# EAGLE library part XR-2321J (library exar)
V.23/V.21 MODEM
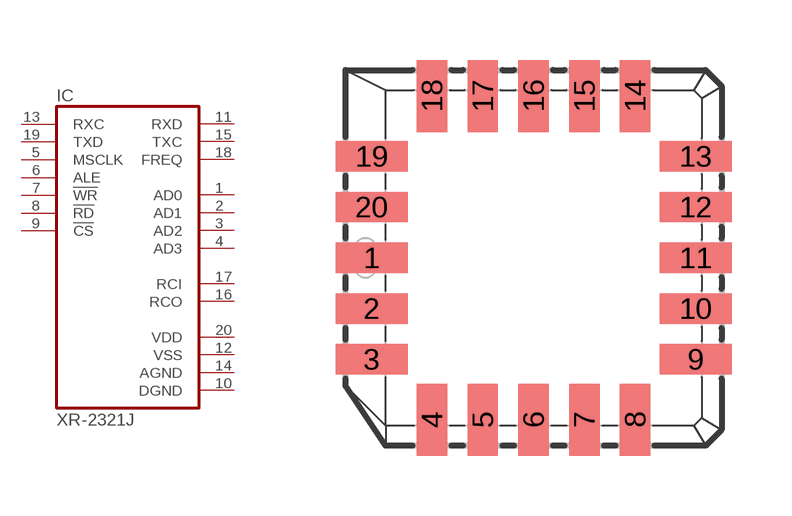
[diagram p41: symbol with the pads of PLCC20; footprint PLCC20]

Designator prefix IC

## XR-2321J (OC_FARNELL: unknown; OC_NEWARK: unknown)  [PLCC20]
1  AD0
2  AD1
3  AD2
4  AD3
5  MSCLK  in
6  ALE  in
7  !WR  in
8  !RD  in
9  !CS  in
10  DGND  pwr
11  RXD  out
12  VSS  pwr
13  RXC  in
14  AGND  pwr
15  TXC  out
16  RCO
17  RCI
18  FREQ  out
19  TXD  in
20  VDD  pwr

## Footprint PLCC20 (pad centres in mm)
Plastic Leaded Chip Carrier
smd 1.8 x 0.76: 1 -4.05,0; 2 -4.05,-1.27; 3 -4.05,-2.54; 9 4.05,-2.54; 10 4.05,-1.27; 11 4.05,0; 12 4.05,1.27; 13 4.05,2.54; 19 -4.05,2.54; 20 -4.05,1.27
smd 0.76 x 1.8: 4 -2.54,-4.05; 5 -1.27,-4.05; 6 0,-4.05; 7 1.27,-4.05; 8 2.54,-4.05; 14 2.54,4.05; 15 1.27,4.05; 16 0,4.05; 17 -1.27,4.05; 18 -2.54,4.05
